FUNCTION_BLOCK FB102
TITLE =Get Version
//*****************************************************************************
//* maxon motor ag
//* R&D
//* all rights reserved
//*****************************************************************************
//* Summary:  Reads the Hardware-, Software-, Application Version and
//*           Application Number
//*
//* Remarks:
//*
//* Created under: STEP7 REV5.2+SP1
//*****************************************************************************
//* History:
//* 19.05.2004 | INA   first release
//*
//*
//*****************************************************************************
//

AUTHOR:INA
FAMILY:Utilitie
NAME:GetVersi
VERSION:00.01


VAR_INPUT

Read : BOOL //A rising edge start the command

  NodeID : BYTE //Adress of the maxon device

END_VAR
VAR_OUTPUT
  Done : BOOL //Data valid flag is TRUE if data were available

  Err : BOOL //Error flag is TRUE if an Error has occured, see ErrNo for more details

  ErrNo : DINT //Contains detailed error information

  HardwareVersion : WORD //Hardware Version

  SoftwareVersion : WORD //Software Version

  ApplicationNumber : WORD //Application Number

  ApplicationVersion : WORD //Application Version

END_VAR
VAR
  xEdgeMerker : BOOL //Edge Merker

  xEdgeFlag : BOOL //Edge Flag

  xStep : INT
END_VAR

BEGIN

NETWORK
TITLE = Activate the service function
//

// SDO Read "Get Version"

       U    #Read
       FP   #xEdgeFlag                   // recognize a positiv edge of the Read signal
       =    #xEdgeMerker                 // and set the xEdgeMerker for one cycle to true

       L    #xStep
       L    0
       ==I
       U    #xEdgeMerker
       SPB  nstp                         // iStep = 1 -> fnc1

       L    #xStep                       // jump list
       SPL  List
       SPA  rdef
       SPA  fnc1
       SPA  fncE
List  :SPA  rdef

rdef  :NOP  0
       R    #Done                        // reset Done
       R    #Err                         // reset Error
       L    0
       T    #xStep                       // iStep = 0
       SPA  end

fnc1  :NOP  0
       CALL FC1
         NodeID:=#NodeID
         Index:=DW#16#00002003
         SubIndex:=DW#16#00000001
         RET_VAL:=#Done
         Err:=#Err
         ErrNo:=#ErrNo

       L    DB219.DBW10
       T    #HardwareVersion

       L    1
       U    #Err
       SPB  fncE

       NOP  0
       CALL FC1
         NodeID:=#NodeID
         Index:=DW#16#00002003
         SubIndex:=DW#16#00000002
         RET_VAL:=#Done
         Err:=#Err
         ErrNo:=#ErrNo

       L    DB219.DBW10
       T    #SoftwareVersion

       L    1
       U    #Err
       SPB  fncE

       NOP  0
       CALL FC1
         NodeID:=#NodeID
         Index:=DW#16#00002003
         SubIndex:=DW#16#00000003
         RET_VAL:=#Done
         Err:=#Err
         ErrNo:=#ErrNo

       L    DB219.DBW10
       T    #ApplicationNumber

       L    1
       U    #Err
       SPB  fncE

       NOP  0
       CALL FC1
         NodeID:=#NodeID
         Index:=DW#16#00002003
         SubIndex:=DW#16#00000004
         RET_VAL:=#Done
         Err:=#Err
         ErrNo:=#ErrNo

       L    DB219.DBW10
       T    #ApplicationVersion

fncE  :NOP  0
       L    0
       T    #xStep
       SPA  end

nstp  :NOP  0
       L    #xStep
       INC            1
       T    #xStep

end   :NOP  0
END_FUNCTION_BLOCK
